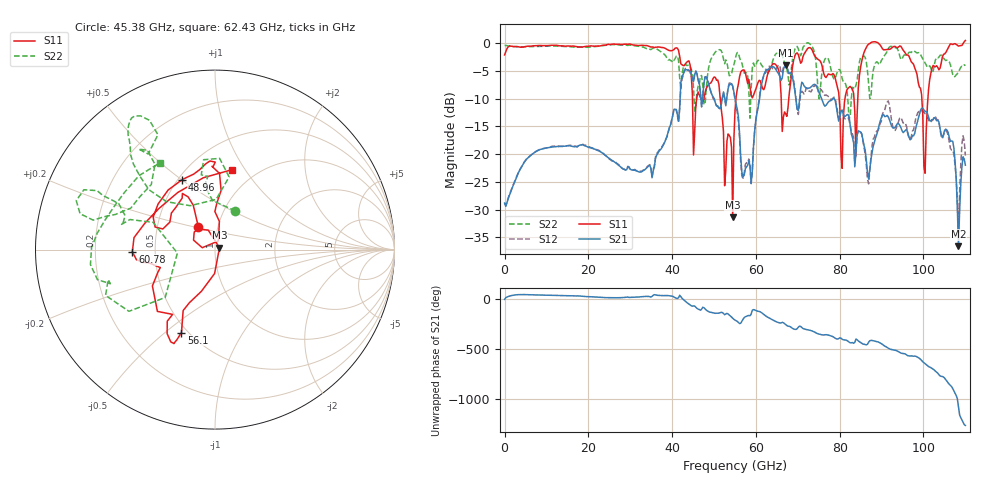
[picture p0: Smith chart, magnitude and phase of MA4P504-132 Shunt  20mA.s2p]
!Keysight Technologies,N5247B,US61255204,A.15.70.20
!Date: Friday, October 21, 2022 14:58:44
!Correction: S11(C  4-Port  )
!S31(C  4-Port  )
!S13(C  4-Port  )
!S33(C  4-Port  )
!S2P File: Measurements: S11, S31, S13, S33:
# Hz S  dB  R 50
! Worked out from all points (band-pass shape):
!   401 points, 10 MHz to 110 GHz, reference 50 ohm
!   highest |S21| = -3.95 dB at 67.1 GHz (marker M1); lowest = -36.6 dB at 108.4 GHz (marker M2)
!   |S21| within 3 dB of the highest: 42.14 GHz to 46.33 GHz (4.199 GHz wide, 9.49 % of centre); 61.5 GHz to 68.92 GHz (7.422 GHz wide, 11.4 % of centre)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
!   lowest |S11| = -31.4 dB at 54.46 GHz (marker M3), VSWR 1.06, Z = 52.6 + j1.06 ohm
!   |S11| at or under -10 dB: 51.48 GHz to 55.24 GHz (3.763 GHz wide, 7.05 % of centre); 66.03 GHz to 67.84 GHz (1.815 GHz wide, 2.71 % of centre); 79.86 GHz to 81.27 GHz (1.402 GHz wide, 1.74 % of centre)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
!   |S22| runs from -13.7 to 0.0 dB; largest |S21 - S12| = 0.24
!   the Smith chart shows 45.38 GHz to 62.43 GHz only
!   S11 on the Smith chart (normalised r, x): 45.38 GHz: 0.80, +0.21; 48.96 GHz: 0.53, +0.50; 56.1 GHz: 0.46, -0.57; 60.78 GHz: 0.37, -0.01; 62.43 GHz: 0.78, +0.87
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1e7  -2.16 -179.8  -28.81 -7.2  -28.82 -6.5  -0.46 -180.0
1.843332e10  -0.76 117.9  -18.33 25.4  -18.35 25.5  -0.74 124.5
3.685665e10  -0.74 115.3  -19.48 32.6  -19.32 32.6  -1.34 122.2
4.373102e10  -3.31 17.1  -4.93 -44.9  -4.77 -42.8  -4.04 81.4
4.538088e10  -16.00 125.9  -5.69 -73.4  -5.62 -72.6  -12.25 62.2
4.895555e10  -7.32 115.1  -8.05 -133.5  -7.99 -131.7  -3.63 133.6
5.445505e10  -31.39 21.8  -7.76 164.5  -7.84 163.7  -4.61 160.6
5.5005e10  -12.24 -108.1  -9.96 146.4  -10.20 144.6  -3.12 166.4
5.61049e10  -6.05 -112.0  -16.43 111.0  -17.36 114.7  -2.68 153.4
6.077948e10  -6.73 -178.5  -10.51 -127.2  -10.08 -122.6  -3.25 179.1
6.242932e10  -6.85 78.1  -4.91 -174.9  -5.15 -168.5  -4.84 122.3
6.462912e10  -3.83 16.2  -4.61 133.8  -4.73 155.2  -2.10 62.5
6.71039e10  -12.76 -41.3  -3.95 101.4  -3.63 101.8  -4.31 45.6
7.342832e10  -1.29 138.8  -7.71 37.6  -8.41 36.0  -0.67 108.5
8.112762e10  -10.66 -28.9  -13.29 -51.7  -13.62 -52.4  -7.13 -125.3
8.525225e10  -3.33 39.1  -16.32 -86.2  -16.42 -84.8  -2.48 -23.2
9.185165e10  -1.15 91.0  -13.79 -140.5  -11.14 -134.5  -0.76 83.8
9.872602e10  -7.05 150.1  -13.66 131.9  -12.45 131.4  -1.75 176.9
1.003759e11  -23.45 -21.4  -12.30 70.2  -12.73 72.2  -3.62 -156.0
1.036756e11  -4.83 -33.8  -14.21 -39.4  -14.09 -36.1  -2.57 -89.7
1.083502e11  -0.58 22.2  -36.57 -3.4  -34.15 2.4  -5.17 -5.2
1.1e11  0.44 54.4  -22.00 172.3  -20.25 174.4  -4.09 16.5
